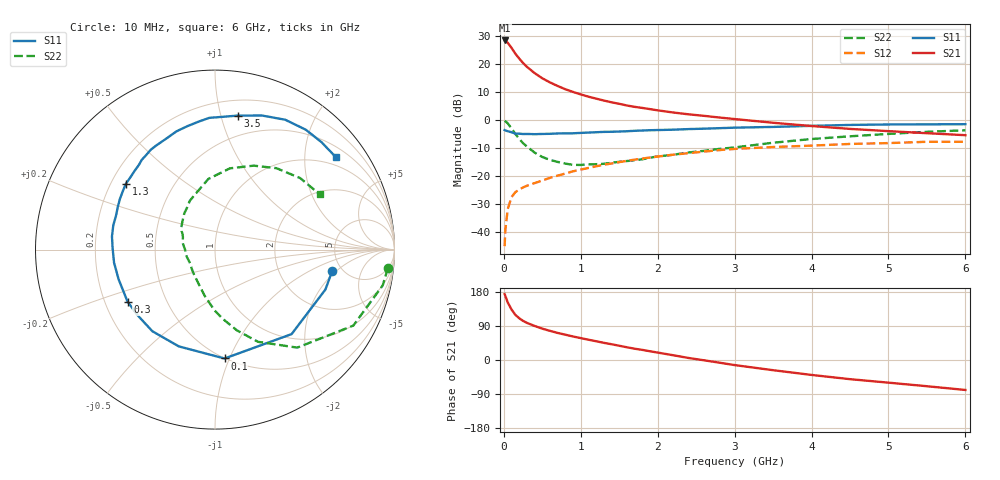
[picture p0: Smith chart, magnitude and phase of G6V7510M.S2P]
! SIEMENS Small Signal Semiconductors
! BFG193
! Si NPN RF Bipolar Junction Transistor in SOT223
! VCE = 0.75 V  IC = 10 mA
! Common Emitter S-Parameters:  August  1996
# GHz  S  MA  R  50
!  f  S11  S21  S12  S22
! GHz  MAG  ANG  MAG  ANG  MAG  ANG  MAG  ANG
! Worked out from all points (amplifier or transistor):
!   36 points, 10 MHz to 6 GHz, reference 50 ohm
!   highest |S21| = 28.5 dB at 10 MHz (marker M1)
!   |S21| within 3 dB of that: start of sweep to 108.2 MHz
!   unconditionally stable (mu >= 1): 810.2 MHz to 3.959 GHz
!   at 250 MHz: K = 0.55, MSG = 22.2 dB, |S12| = -24.0 dB
!   at 1.4 GHz: K = 1.09, MAG = 9.1 dB, |S12| = -15.5 dB
!   at 6 GHz: K = 0.98, MSG = 1.2 dB, |S12| = -7.7 dB
!   S11 on the Smith chart (normalised r, x): 10 MHz: 4.16, -1.77; 100 MHz: 0.50, -0.96; 300 MHz: 0.30, -0.25; 1.3 GHz: 0.26, +0.31; 3.5 GHz: 0.32, +1.13; 6 GHz: 0.76, +2.77
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0.01  0.664 -10.3  26.59 173.9  0.0056 89.2  0.969 -6.1
0.02  0.6541 -19.9  26.25 169.0  0.011 83.7  0.9553 -12.1
0.05  0.6354 -47.8  24.2 152.1  0.0256 68.6  0.8792 -28.8
0.1  0.609 -85.0  19.58 133.2  0.0422 56.2  0.7128 -50.0
0.15  0.5757 -110.5  15.4 119.0  0.0517 48.4  0.5668 -65.0
0.2  0.5733 -127.5  12.62 110.2  0.0577 45.0  0.4654 -74.9
0.25  0.5655 -139.7  10.51 103.2  0.0628 43.2  0.3874 -83.7
0.3  0.567 -149.2  8.991 97.9  0.0674 43.0  0.338 -90.5
0.4  0.562 -162.8  6.936 89.9  0.075 43.1  0.2637 -102.6
0.5  0.5671 -172.7  5.6 82.7  0.0835 43.5  0.2198 -112.9
0.6  0.5704 179.4  4.724 76.9  0.0932 44.3  0.1952 -122.1
0.7  0.5787 172.7  4.078 71.4  0.102 44.5  0.1794 -131.5
0.8  0.5826 166.6  3.571 66.7  0.1115 43.8  0.1673 -141.0
1.1  0.6004 151.9  2.63 53.5  0.14 42.0  0.162 -164.8
1.3  0.6173 143.6  2.244 45.3  0.1597 39.5  0.1661 -179.4
1.7  0.6455 129.2  1.731 29.8  0.1968 33.1  0.1919 158.7
2.2  0.6759 113.5  1.372 12.6  0.2414 22.7  0.2406 138.9
2.8  0.7194 97.1  1.116 -7.0  0.2919 9.8  0.3064 117.2
3.5  0.7574 80.3  0.899 -26.9  0.3316 -7.0  0.3952 95.4
4.5  0.8225 61.6  0.698 -50.6  0.3761 -25.9  0.5148 65.3
5.5  0.8428 45.3  0.585 -69.2  0.4109 -48.0  0.6196 40.0
6  0.8478 37.4  0.539 -79.1  0.4107 -60.7  0.6594 27.9
